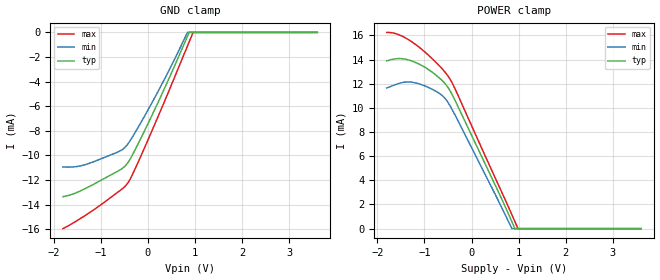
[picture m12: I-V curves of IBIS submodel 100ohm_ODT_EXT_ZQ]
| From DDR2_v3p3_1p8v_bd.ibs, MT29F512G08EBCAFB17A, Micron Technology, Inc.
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| SUBMODEL 100ohm_ODT_EXT_ZQ
[Submodel]   100ohm_ODT_EXT_ZQ
Submodel_type  Dynamic_clamp
[GND Clamp]
|   Voltage   I(typ)   I(min)   I(max)
-1.8V     -13.36mA   -10.95mA   -15.96mA
-1.502V   -13.01mA   -10.91mA   -15.31mA
-1.159V   -12.37mA   -10.54mA   -14.46mA
-582mV    -11.17mA   -9.627mA   -12.84mA
-504.5mV  -10.95mA   -9.421mA   -12.6mA
-432.5mV  -10.65mA   -9.124mA   -12.29mA
-353mV    -10.16mA   -8.68mA    -11.78mA
-230mV    -9.26mA    -7.892mA   -10.78mA
196.5mV   -5.877mA   -4.967mA   -7.048mA
704.5mV   -1.542mA   -1.114mA   -2.391mA
878mV     0A         NA         NA
3.6V      0A         0A         0A
[POWER Clamp]
|   Voltage   I(typ)   I(min)   I(max)
-1.8V     13.88mA    11.65mA    16.24mA
-1.491V   14.07mA    12.07mA    15.97mA
-1.303V   13.92mA    12.14mA    15.56mA
-1.15V    13.69mA    12.03mA    15.13mA
-953mV    13.27mA    11.76mA    14.5mA
-690mV    12.5mA     11.22mA    13.5mA
-516.5mV  11.78mA    10.55mA    12.73mA
-445mV    11.34mA    10.1mA     12.3mA
-335mV    10.5mA     9.295mA    11.45mA
805mV     1.04mA     424.9uA    1.619mA
922mV     0A         NA         NA
3.6V      0A         0A         0A
